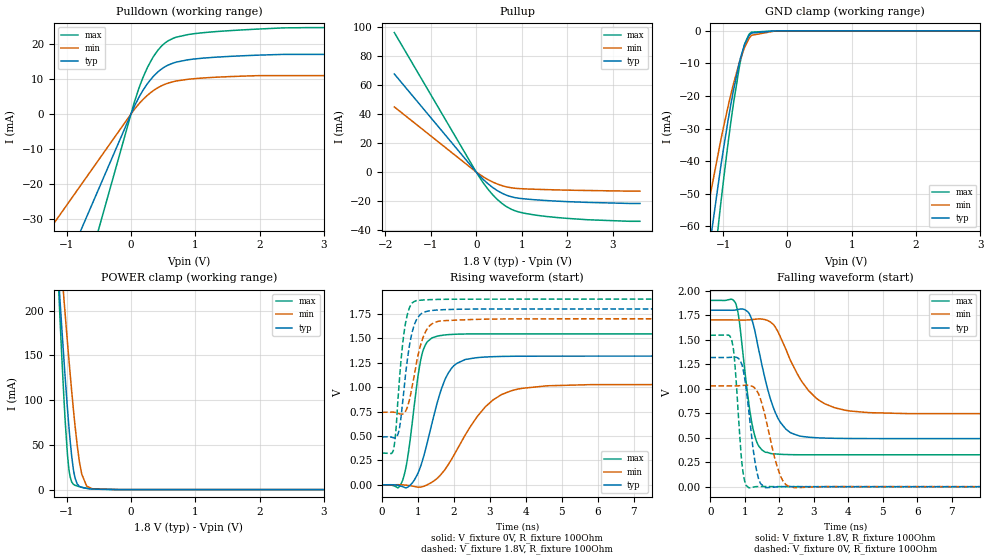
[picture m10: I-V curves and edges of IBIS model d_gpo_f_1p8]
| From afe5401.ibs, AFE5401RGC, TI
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|   d_gpo_f_1p8 Model
[Model]   d_gpo_f_1p8
Model_type   3-state
Polarity   Non-Inverting
Vmeas = 0.9
Vref = 0
Cref = 5pF
Rref = 100
|   typ   min   max
|   (nom PVT)   (fast PVT)   (slow PVT)
C_comp   1.720e-12   1.693e-12   1.765e-12
| Where nom  PVT is Nominal Process, 1.8V, 27C
|   Fast PVT is Strong Process,  1.9V, -40C
|   Slow PVT is Weak Process,   1.7V, 125C
[Voltage Range]   1.8   1.7   1.9
|Junction Temperature
[Temperature Range]   27   125   -40
[Pullup Reference]   1.8   1.7   1.9
[Pulldown Reference]   0   0   0
[Power Clamp Reference]   1.8   1.7   1.9
[GND Clamp Reference]   0   0   0
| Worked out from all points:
|   slope of the pulldown table from 0 to 0.27 V, typ, clamps not added: 29.9 ohm
|   slope of the pullup table from 0 to 0.27 V, typ, clamps not added: 32.3 ohm
|   GND clamp passes 1 mA (typ) near -0.58 V on its own axis
|   POWER clamp passes 1 mA (typ) near -0.65 V on its own axis
|   falling waveform, V_fixture 1.8V, R_fixture 100Ohm: 20-80 % time 567ps typ, 926ps min, 334ps max; typ from 1.8 V to 0.49 V
|   rising waveform, V_fixture 0V, R_fixture 100Ohm: 20-80 % time 589ps typ, 1.11ns min, 329ps max; typ from 0 V to 1.32 V
|   rising waveform, V_fixture 1.8V, R_fixture 100Ohm: 20-80 % time 277ps typ, 341ps min, 221ps max; typ from 0.49 V to 1.8 V
|   falling waveform, V_fixture 0V, R_fixture 100Ohm: 20-80 % time 274ps typ, 423ps min, 181ps max; typ from 1.32 V to 0 V
[Pulldown]
|   Voltage   I(typ)   I(min)   I(max)
-1.8V     -76.98mA   -47.08mA   -118.3mA
-82.4mV   -3.524mA   -2.155mA   -5.414mA
46.2mV    1.923mA    1.16mA     3.004mA
120.9mV   4.691mA    2.853mA    7.272mA
250.2mV   8.566mA    5.277mA    13.13mA
337.5mV   10.59mA    6.572mA    16.12mA
419.2mV   12.08mA    7.548mA    18.3mA
576.9mV   14.01mA    8.848mA    20.97mA
888.5mV   15.54mA    9.948mA    22.77mA
1.329V    16.29mA    10.54mA    23.63mA
2.367V    17.08mA    11mA       24.68mA
3.6V      17.08mA    11mA       24.75mA
[GND Clamp]
|   Voltage   I(typ)   I(min)   I(max)
-1.8V     -248.3mA   -141.1mA   -369.9mA
-1.355V   -87.44mA   -67.03mA   -111.4mA
-1.264V   -73.66mA   -56.96mA   -94.03mA
-1.251V   -71.69mA   -55.52mA   -91.53mA
-1.042V   -42.28mA   -34.06mA   -53.8mA
-880.4mV  -22.58mA   -19.54mA   -27.97mA
-749.3mV  -9.832mA   -9.781mA   -11.19mA
-665.7mV  -4.149mA   -5.031mA   -4.024mA
-601.5mV  -1.56mA    -2.475mA   -1.184mA
-559.8mV  -686.7uA   -1.383mA   -422uA
-180mV    0A         -265.4nA   0A
3.6V      0A         0A         0A
[Pullup]
|   Voltage   I(typ)   I(min)   I(max)
-1.8V     67.66mA    44.92mA    96.24mA
37.7mV    -1.323mA   -861.2uA   -1.926mA
262.8mV   -8.19mA    -5.306mA   -12mA
442.3mV   -12.38mA   -7.986mA   -18.27mA
574.2mV   -14.73mA   -9.461mA   -21.88mA
682.2mV   -16.19mA   -10.35mA   -24.2mA
898mV     -17.92mA   -11.34mA   -27.21mA
1.47V     -19.54mA   -12.07mA   -30.41mA
2.454V    -20.97mA   -12.76mA   -32.94mA
3.6V      -21.69mA   -13.18mA   -34.01mA
[POWER Clamp]
|   Voltage   I(typ)   I(min)   I(max)
-1.8V     1.059A     958.6mA    1.413A
-1.135V   246.4mA    298.1mA    240mA
-1.094V   200.8mA    260.2mA    176.2mA
-1.04V    142.2mA    210.6mA    97.99mA
-986.8mV  89.35mA    163.6mA    38.2mA
-946.9mV  54.97mA    129.9mA    14.38mA
-887.4mV  18.91mA    83.53mA    5.518mA
-834.4mV  6.082mA    48.36mA    3.917mA
-766.4mV  2.485mA    17.42mA    2.633mA
-689.9mV  1.369mA    3.936mA    1.474mA
-601.1mV  588.9uA    933.8uA    530.1uA
3.6V      0A         0A         0A
[Ramp]
R_load = 100
|   typ   min   max
dV/dt_r   0.790309/5.87579e-10   0.616855/1.10239e-09   0.92655/3.28967e-10
dV/dt_f   0.785852/5.66334e-10   0.574603/9.18269e-10   0.944751/3.3414e-10
[Falling Waveform]
V_fixture = 1.8V
V_fixture_min = 1.7V
V_fixture_max = 1.9V
R_fixture = 100Ohm
|   Time   V(typ)   V(min)   V(max)
0s        1.8V       1.7V       1.9V
740ps     1.802V     1.7V       1.865V
840ps     1.81V      1.699V     1.693V
1.22ns    1.686V     1.704V     622.4mV
1.595ns   1.089V     1.703V     351.6mV
1.955ns   702.5mV    1.585V     332.8mV
2.31ns    554mV      1.299V     327mV
3.07ns    499.6mV    902.8mV    325.5mV
3.915ns   492mV      779.5mV    325.5mV
14.99ns   490.2mV    742.3mV    325.4mV
[Rising Waveform]
V_fixture = 0V
V_fixture_min = 0V
V_fixture_max = 0V
R_fixture = 100Ohm
|   Time   V(typ)   V(min)   V(max)
0s        983.6pV    73.44nV    402.5pV
565ps     -17.99mV   -130uV     39.24mV
725ps     -21.47mV   -6.043mV   307.6mV
1.105ns   224.9mV    -20.27mV   1.326V
1.535ns   839.4mV    66.74mV    1.521V
1.775ns   1.096V     169.1mV    1.535V
2.085ns   1.243V     359.1mV    1.542V
2.885ns   1.308V     801.3mV    1.544V
3.76ns    1.316V     977.9mV    1.544V
14.99ns   1.317V     1.028V     1.544V
[Rising Waveform]
V_fixture = 1.8V
V_fixture_min = 1.7V
V_fixture_max = 1.9V
R_fixture = 100Ohm
|   Time   V(typ)   V(min)   V(max)
0s        490.2mV    742.3mV    325.4mV
315ps     481.2mV    743.4mV    353.4mV
385ps     482.3mV    739.2mV    557.9mV
465ps     546.3mV    729.6mV    983.9mV
660ps     1.151V     757.4mV    1.667V
800ps     1.499V     933.3mV    1.839V
945ps     1.679V     1.219V     1.883V
1.225ns   1.773V     1.577V     1.893V
1.595ns   1.79V      1.675V     1.897V
14.99ns   1.8V       1.7V       1.9V
[Falling Waveform]
V_fixture = 0V
V_fixture_min = 0V
V_fixture_max = 0V
R_fixture = 100Ohm
|   Time   V(typ)   V(min)   V(max)
0s        1.317V     1.028V     1.544V
620ps     1.32V      1.027V     1.494V
715ps     1.322V     1.028V     1.241V
930ps     1.227V     1.032V     199.7mV
1.125ns   742.2mV    1.034V     -11.14mV
1.3ns     246.7mV    1.001V     -153.4uV
1.45ns    36.86mV    898.9mV    1.955mV
2.03ns    367.2uV    112.6mV    724.2uV
2.43ns    1.181mV    -9.648mV   366uV
14.99ns   29.03nV    647.2nV    -5.52nV
